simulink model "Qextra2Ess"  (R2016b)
settings: Solver=ode45  StartTime=0.0  StopTime=100  RelTol=1e-6  EnableMultiTasking=on
libraries: simulink x2

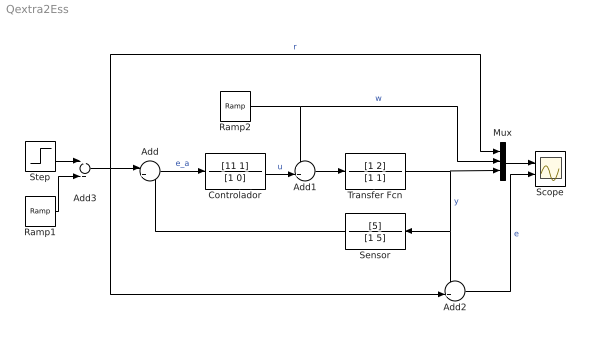
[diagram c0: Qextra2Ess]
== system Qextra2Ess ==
  Add : Sum  Inputs=|+-
  Add1 : Sum  Inputs=++|
  Add2 : Sum  Inputs=-+|
  Add3 : Sum
  Controlador : TransferFcn  Numerator=[11 1]  Denominator=[1 0]
  Mux : Mux  Inputs=3
  Ramp1 : simulink/Sources/Ramp  slope=5/3  start=2  X0=0
  Ramp2 : simulink/Sources/Ramp  slope=-1/4  start=1  X0=0
  Scope : Scope  NumInputPorts=2
  Sensor : TransferFcn  Numerator=[5]  Denominator=[1 5]
  Step : Step  Time=0  After=2  SampleTime=0
  Transfer Fcn : TransferFcn  Numerator=[1 2]  Denominator=[1 1]
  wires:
  Add3/1 -> Mux/1, Add2/2, Add/1  "r"
  Transfer Fcn/1 -> Add2/1, Sensor/1, Mux/3  "y"
  Add/1 -> Controlador/1  "e_a"
  Mux/1 -> Scope/1
  Add2/1 -> Scope/2  "e"
  Sensor/1 -> Add/2
  Add1/1 -> Transfer Fcn/1
  Controlador/1 -> Add1/2  "u"
  Step/1 -> Add3/1
  Ramp1/1 -> Add3/2
  Ramp2/1 -> Mux/2, Add1/1  "w"
